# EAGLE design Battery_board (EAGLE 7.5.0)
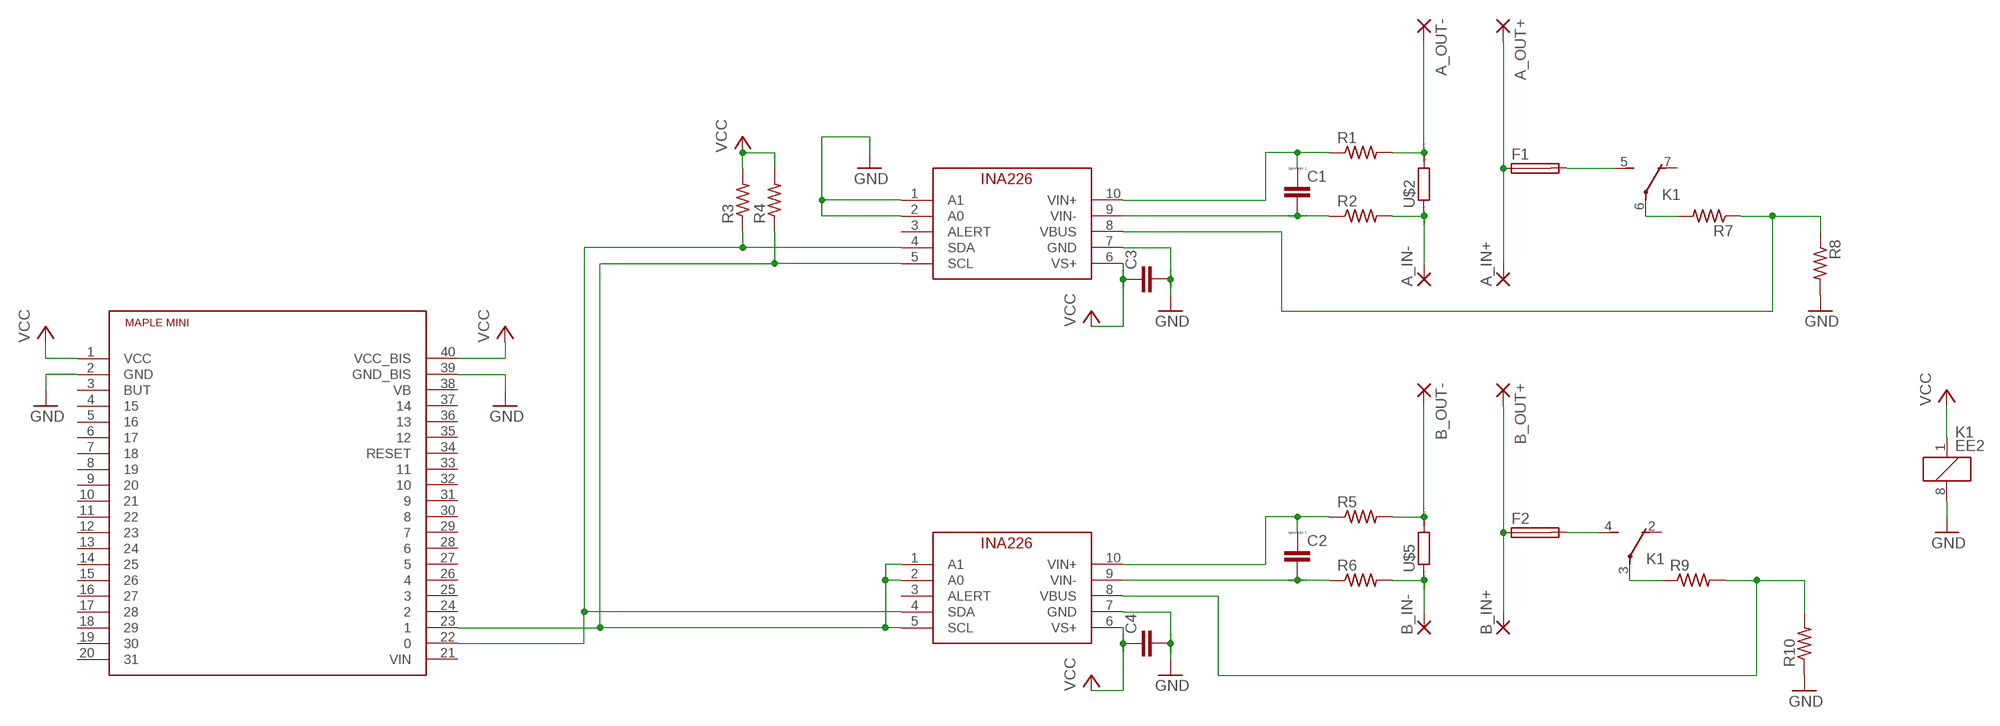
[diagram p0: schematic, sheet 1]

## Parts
A_IN+  WIREPAD4,16O1,6  [4,16O1,6]
A_IN-  WIREPAD4,16O1,6  [4,16O1,6]
A_OUT+  WIREPAD4,16O1,6  [4,16O1,6]
A_OUT-  WIREPAD4,16O1,6  [4,16O1,6]
B_IN+  WIREPAD4,16O1,6  [4,16O1,6]
B_IN-  WIREPAD4,16O1,6  [4,16O1,6]
B_OUT+  WIREPAD4,16O1,6  [4,16O1,6]
B_OUT-  WIREPAD4,16O1,6  [4,16O1,6]
C1  CC0603  [C0603]
C2  CC0603  [C0603]
C3  CC0603  [C0603]
C4  CC0603  [C0603]
F1  TE5  [TE5]
F2  TE5  [TE5]
K1  EE2  [EE2-5NU]
R1  R-US_R0603  [R0603]
R2  R-US_R0603  [R0603]
R3  R-US_R0603  [R0603]
R4  R-US_R0603  [R0603]
R5  R-US_R0603  [R0603]
R6  R-US_R0603  [R0603]
R7  R-US_R1206  [R1206]
R8  R-US_R1206  [R1206]
R9  R-US_R1206  [R1206]
R10  R-US_R1206  [R1206]
U$1  INA226  [MSOP10]
U$2  R_SHUNT_2526  [R2526]
U$3  MAPLE_MINI  [DIL40_MAPLE]
U$4  INA226  [MSOP10]
U$5  R_SHUNT_2526  [R2526]

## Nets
GND: C3.2 C4.2 K1.8 R8.2 R10.1 U$1.1(A1) U$1.2(A0) U$1.7(GND) U$3.2(GND) U$3.39(GND_BIS) U$4.7(GND)
N$1: R4.1 U$1.5(SCL) U$3.23 U$4.1(A1) U$4.2(A0) U$4.5(SCL)
N$2: C1.1 R1.1 U$1.10(VIN+)
N$3: C1.2 R2.1 U$1.9(VIN-)
N$4: F1.2 K1.5(3:S)
N$7: A_OUT-.1(P) R1.2 U$2.2
N$8: A_IN-.1(P) R2.2 U$2.1
N$9: A_IN+.1(P) A_OUT+.1(P) F1.1
N$10: F2.2 K1.4(2:S)
N$12: C2.1 R5.1 U$4.10(VIN+)
N$13: C2.2 R6.1 U$4.9(VIN-)
N$16: R3.1 U$1.4(SDA) U$3.22 U$4.4(SDA)
N$18: B_OUT-.1(P) R5.2 U$5.2
N$19: B_IN-.1(P) R6.2 U$5.1
N$20: B_IN+.1(P) B_OUT+.1(P) F2.1
N$21: K1.3(2:P) R9.1
N$22: R9.2 R10.2 U$4.8(VBUS)
N$23: K1.6(3:P) R7.2
N$24: R7.1 R8.1 U$1.8(VBUS)
VCC: C3.1 C4.1 K1.1 R3.2 R4.2 U$1.6(VS+) U$3.1(VCC) U$3.40(VCC_BIS) U$4.6(VS+)
Unconnected: K1.2(2:O) K1.7(3:O) U$1.3(ALERT) U$3.3(BUT) U$3.4 U$3.5 U$3.6 U$3.7 U$3.8 U$3.9 U$3.10 U$3.11 U$3.12 U$3.13 U$3.14 U$3.15 U$3.16 U$3.17 U$3.18 U$3.19 U$3.20 U$3.21(VIN) U$3.24 U$3.25 U$3.26 U$3.27 U$3.28 U$3.29 U$3.30 U$3.31 U$3.32 U$3.33 U$3.34(RESET) U$3.35 U$3.36 U$3.37 U$3.38(VB) U$4.3(ALERT)

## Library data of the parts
A_IN+ A_IN- A_OUT+ A_OUT- B_IN+ B_IN- B_OUT+ B_OUT- = wirepad:WIREPAD: Wire PAD connect wire on PCB
C1-C4 = eagle-ltspice:C: CAPACITOR, European symbol; SPICEMODEL: NONE; SPICEPREFIX: C
F1 F2 = fuse:TE5: FUSE; OC_FARNELL: unknown; OC_NEWARK: unknown
K1 = CUSTOM:EE2: Compact & Slim 2 Form C Non-polarized Relay NAiS Source: http://www.mew-europe.com/.. en_ds_61011_0000.pdf
R1-R10 = resistor:R-US_: RESISTOR, American symbol
U$1 U$4 = CUSTOM:INA226: INA226
U$2 U$5 = CUSTOM:R_SHUNT_2526
U$3 = CUSTOM:MAPLE_MINI

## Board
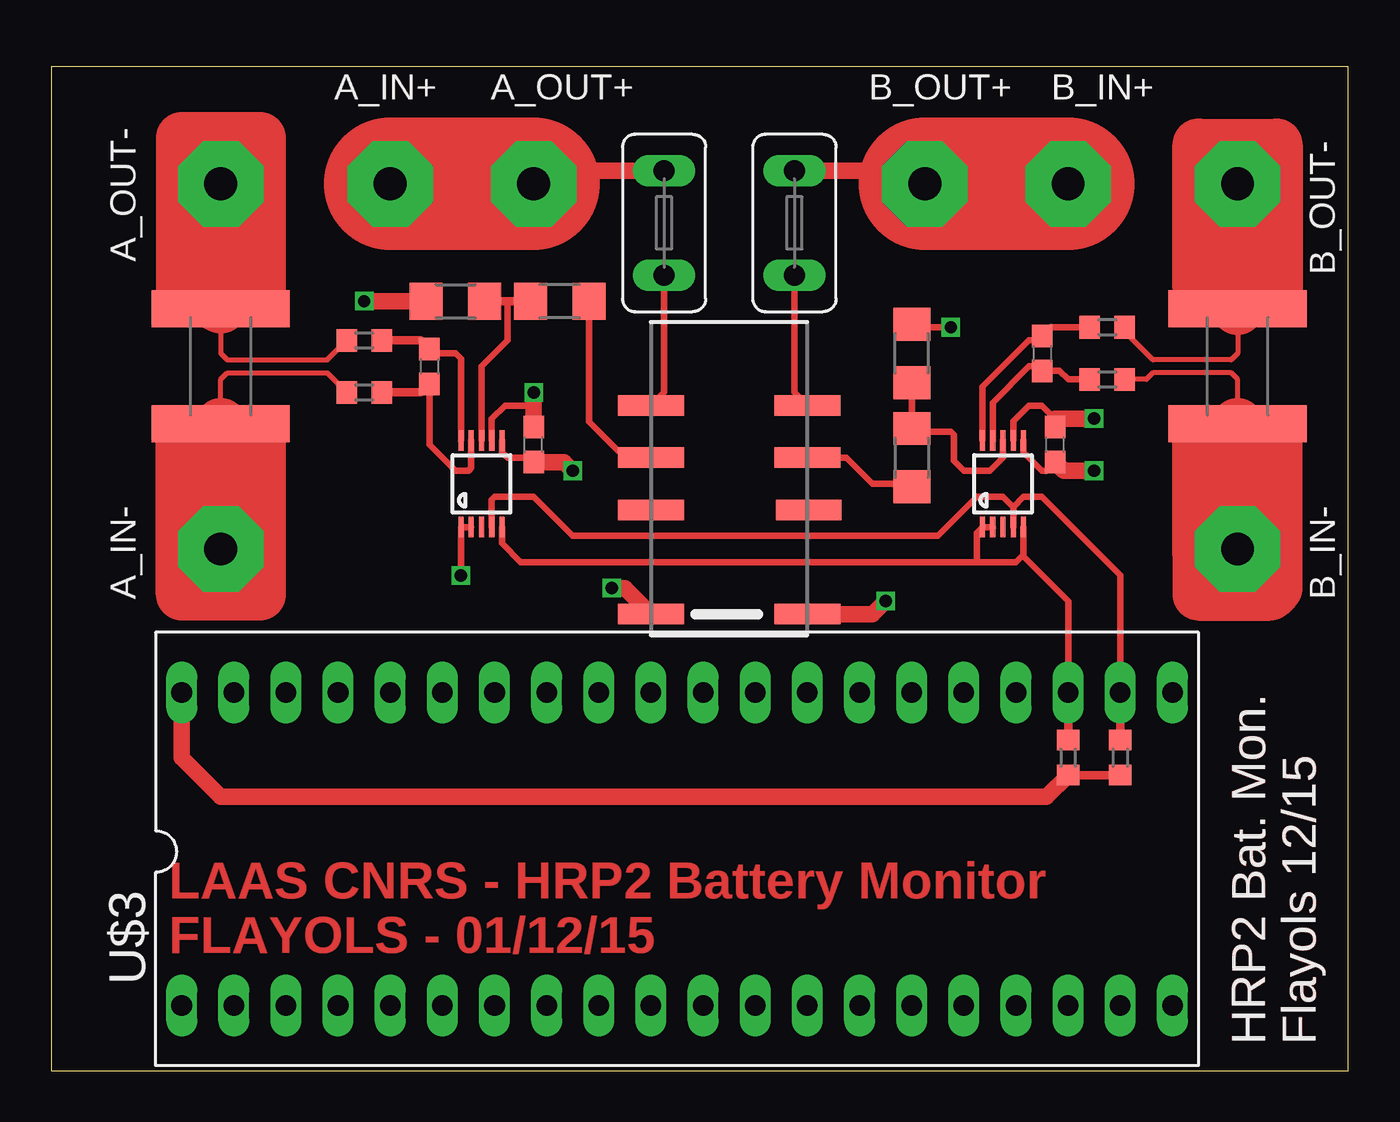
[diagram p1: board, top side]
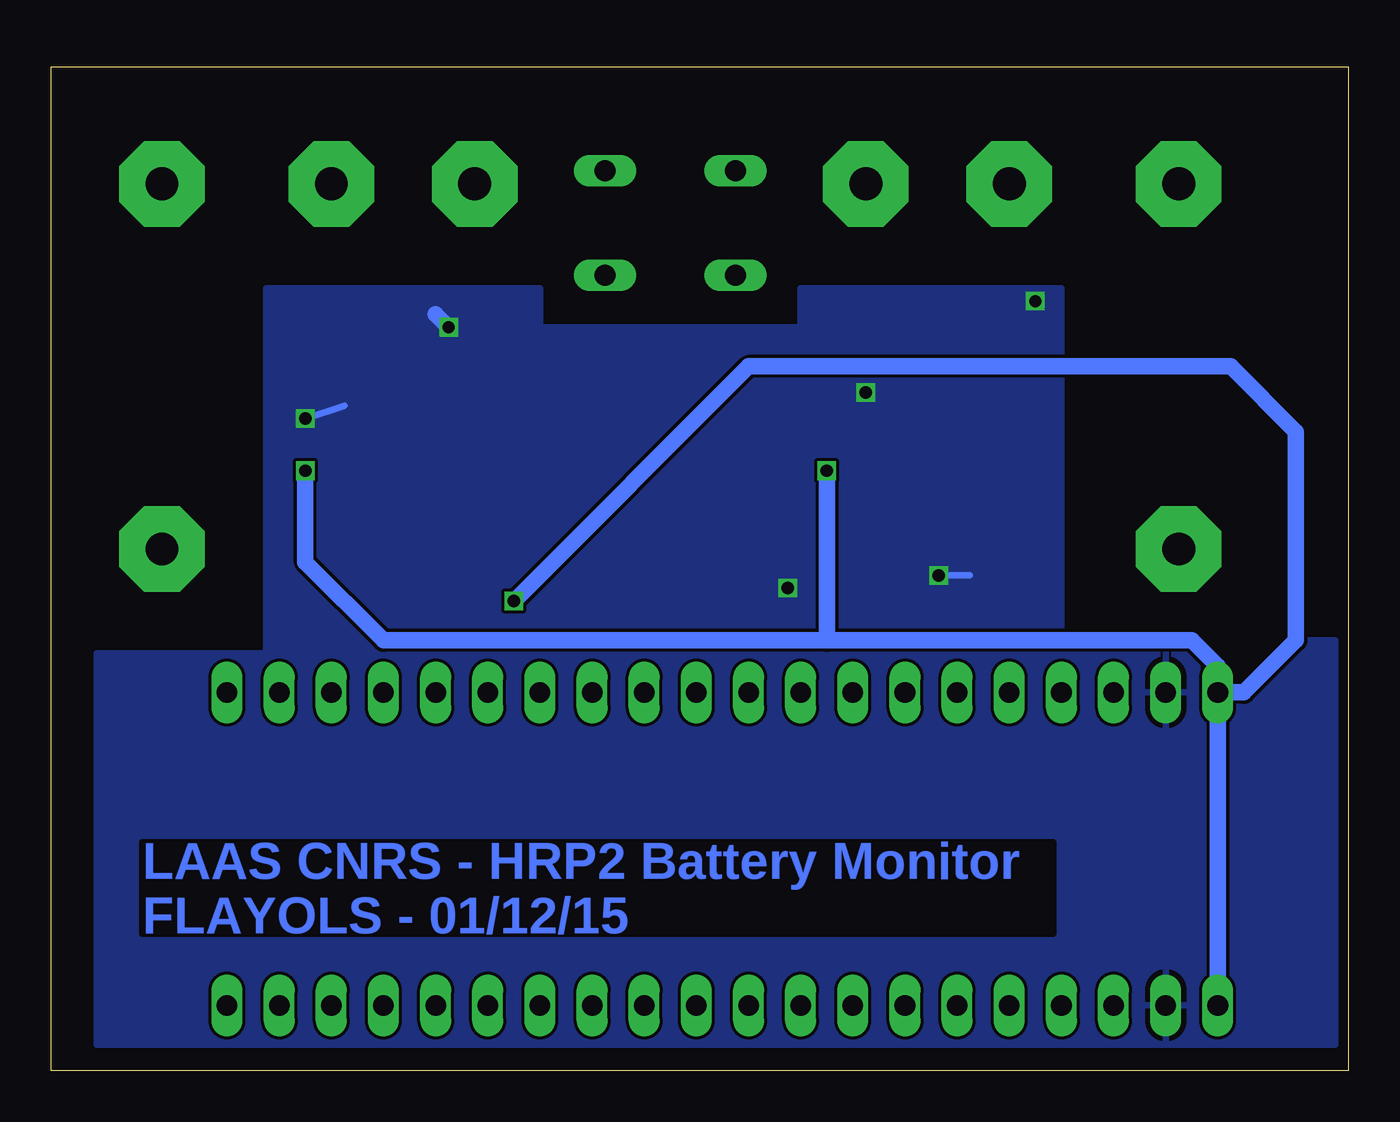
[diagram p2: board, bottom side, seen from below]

Size 63.17 x 48.88 mm. Coordinates in mm from the lower left corner, seen from the top.
Outline: 0,0 63.17,0 63.17,48.88 0,48.88 0,0
Copper layers (1*16): Top 0.035mm / dielectric 1.5mm / Bottom 0.035mm
Design rules "SeeedStudio_2layer_DRU_no_angle_20140221": minimum track width 6mil, minimum drill 12mil, track to track 6mil, track to pad 6mil, pad to pad 6mil, via to via 6mil, smd to smd 0mil, copper to edge 10mil, drill to drill 10mil, minimum pad ring 10mil, minimum via ring 6mil, stop-mask expansion 2mil, vias tented up to drill 100mil, thermal gap 10mil

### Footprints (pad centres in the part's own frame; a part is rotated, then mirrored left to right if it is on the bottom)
4,16O1,6 = drill 1.6 pad 4.166 octagon: 1 0,0
C0603 = smd 1.1 x 1: 1 -0.85,0; 2 0.85,0
TE5 = drill 1.016 long: 1 -2.54,0; 2 2.54,0
EE2-5NU = smd 1 x 3.2: 1 -5.08,-5.08; 2 0,-5.14; 3 2.54,-5.08; 4 5.08,-5.08; 5 5.08,2.54; 6 2.54,2.54; 7 0,2.54; 8 -5.08,2.54
R0603 = smd 1 x 1.1: 1 -0.85,0; 2 0.85,0
R1206 = smd 1.6 x 1.803: 1 -1.422,0; 2 1.422,0
MSOP10 = smd 0.25 x 1: 1 -1,-2.113; 2 -0.5,-2.113; 3 0,-2.113; 4 0.5,-2.113; 5 1,-2.113; 6 1,2.113; 7 0.5,2.113; 8 0,2.113; 9 -0.5,2.113; 10 -1,2.113
R2526 = smd 1.8 x 6.731: 1 -2.8,0; 2 2.8,0
DIL40_MAPLE = drill 1 long: 1 -24.13,-7.62; 2 -21.59,-7.62; 3 -19.05,-7.62; 4 -16.51,-7.62; 5 -13.97,-7.62; 6 -11.43,-7.62; 7 -8.89,-7.62; 8 -6.35,-7.62; 9 -3.81,-7.62; 10 -1.27,-7.62; 11 1.27,-7.62; 12 3.81,-7.62; 13 6.35,-7.62; 14 8.89,-7.62; 15 11.43,-7.62; 16 13.97,-7.62; 17 16.51,-7.62; 18 19.05,-7.62; 19 21.59,-7.62; 20 24.13,-7.62; 21 24.13,7.62; 22 21.59,7.62; 23 19.05,7.62; 24 16.51,7.62; 25 13.97,7.62; 26 11.43,7.62; 27 8.89,7.62; 28 6.35,7.62; 29 3.81,7.62; 30 1.27,7.62; 31 -1.27,7.62; 32 -3.81,7.62; 33 -6.35,7.62; 34 -8.89,7.62; 35 -11.43,7.62; 36 -13.97,7.62; 37 -16.51,7.62; 38 -19.05,7.62; 39 -21.59,7.62; 40 -24.13,7.62

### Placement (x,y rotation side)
A_IN+  16.51,43.18 0 top
A_IN-  8.25,25.4 270 top
A_OUT+  23.5,43.18 0 top
A_OUT-  8.25,43.18 270 top
B_IN+  49.53,43.18 0 top
B_IN-  57.78,25.4 270 top
B_OUT+  42.55,43.18 0 top
B_OUT-  57.78,43.18 270 top
C1  18.41,34.29 270 top
C2  48.26,34.92 270 top
C3  23.5,30.48 90 top
C4  48.9,30.48 90 top
F1  29.84,41.27 270 top
F2  36.2,41.27 270 top
K1  31.75,27.3 90 top
R1  15.24,35.56 180 top
R2  15.24,33.02 180 top
R3  52.07,15.24 270 top
R4  49.53,15.24 270 top
R5  51.44,36.2 0 top
R6  51.44,33.66 0 top
R7  24.77,37.47 0 top
R8  19.68,37.47 180 top
R9  41.91,29.84 90 top
R10  41.91,34.92 270 top
U$1  20.95,28.57 0 top
U$2  8.25,34.29 90 top
U$3  30.48,10.79 0 top
U$4  46.35,28.57 0 top
U$5  57.78,34.29 90 top

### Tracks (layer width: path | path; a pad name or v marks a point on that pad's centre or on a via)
GND  (via drill 0.6)
  Top 0.305: U$4.7 46.85,31.61 47.62,32.38 48.26,32.38 48.9,31.75 C4.2 | U$1.7 21.45,31.75 22.09,32.38 23.5,32.38 | U$1.2 U$1.1 v19.95,24.11 | R10.1 41.91,36.2 v43.81,36.2
  Top 0.813: R8.2 v15.24,37.47 | 48.9,31.75 v50.8,31.75 | v27.3,23.5 27.94,23.5 K1.8 | C3.2 23.5,32.38 v23.5,33.02
  Bottom 0.305: 48.9,32.38 v50.8,31.75 | v19.95,24.11 19.93,24.13 18.41,24.13
  Bottom 0.813: v43.81,36.2 44.45,36.83
  pour Bottom: 13.97,20.95 13.97,38.1 26.67,38.1 26.67,36.2 39.37,36.2 39.37,38.1 52.7,38.1 52.7,20.32 60.96,20.32 60.96,1.27 0.63,1.27 0.63,20.95
N$1
  Top 0.305: U$1.5 21.95,25.67 22.86,24.77 45.09,24.77 | 45.09,24.77 45.09,26.19 U$4.1 U$4.2 | U$3.23 49.53,22.86 47.35,25.04 47.35,25.13 | U$4.5 47.35,25.13 | 47.35,25.13 46.99,24.77 45.09,24.77
  Top 0.406: U$3.23 R4.1
N$2
  Top 0.305: U$1.10 19.95,34.66 19.68,34.92 18.63,34.92 C1.1
  Top 0.406: R1.1 18,35.56 C1.1
N$3
  Top 0.305: U$1.9 20.45,29.34 20.32,29.21 19.68,29.21 18.41,30.48 C1.2
  Top 0.406: R2.1 18,33.02 C1.2
N$4
  Top 0.305: F1.2 29.84,33.02 K1.5
N$7
  Top 0.254: 8.25,37.15 U$2.2 8.25,34.92 8.57,34.61 13.44,34.61 R1.2
  Top 0.406: 8.25,38.1 10.16,37.09 8.89,37.09 U$2.2 | R1.2 14.39,35.34
  Top 1.778: 10.16,37.78 8.89,38.1 8.89,37.09
  Top 2.54: 6.35,45.4 A_OUT-.1 8.25,37.15 7.62,37.47 6.35,37.47 6.35,45.4 | 10.16,37.78 10.16,45.4 6.35,45.4
N$8
  Top 0.254: U$2.1 8.25,33.66 8.57,33.97 13.44,33.97 R2.2
  Top 0.406: R2.2 14.39,33.23
  Top 2.54: A_IN-.1 6.98,25.4 6.35,23.18 | 6.35,23.18 6.35,31.11 8.25,31.11 | 8.89,30.48 8.25,31.11 | 8.25,31.11 A_IN-.1 | A_IN-.1 10.16,23.18 | 10.16,31.11 10.16,23.18 | 10.16,23.18 6.35,23.18 | 6.35,23.18 8.25,25.08 U$2.1
N$9
  Top 0.813: F1.1 24.13,43.81 A_OUT+.1
  Top 6.452: A_IN+.1 A_OUT+.1
N$10
  Top 0.305: F2.2 36.2,33.02 K1.4
N$12
  Top 0.305: R5.1 48.68,36.2 C2.1 48.05,35.56 47.62,35.56 45.35,33.29 U$4.10
N$13
  Top 0.305: U$4.9 45.85,32.52 47.62,34.29 48.05,34.29 C2.2 49.11,34.08 49.53,33.66 R6.1
N$16
  Top 0.305: U$1.4 21.45,27.8 21.59,27.94 23.5,27.94 25.4,26.04 43.18,26.04 45.09,27.94 46.35,27.94 46.85,27.44 | U$3.22 52.07,24.13 48.26,27.94 47.35,27.94 46.85,27.44 | 46.85,27.44 U$4.4
  Top 0.406: U$3.22 R3.1
N$18
  Top 0.254: 55.88,38.1 57.78,36.2 57.78,34.92 57.47,34.61 53.66,34.61 52.28,35.98 R5.2
  Top 2.54: 55.88,38.1 55.88,45.09 59.69,45.09 59.69,37.78 57.78,40.01 B_OUT-.1 U$5.2
N$19
  Top 0.254: 57.78,31.11 U$5.1 57.78,33.66 57.47,33.97 53.66,33.97 53.34,33.66 R6.2 | 55.88,31.11 56.26,31.49
  Top 2.54: 57.78,24.13 B_IN-.1 57.78,27.62 57.78,29.21 | 57.78,24.13 57.78,23.18 55.88,25.08 | 55.88,25.08 55.88,23.5 | 55.88,23.5 55.88,23.18 59.37,23.18 59.69,23.5 59.69,31.11 57.78,29.21 | 57.78,24.13 57.15,23.5 55.88,23.5 | 55.88,25.08 55.88,31.11 | U$5.1 57.78,29.21
N$20
  Top 0.813: 42.55,44.45 B_OUT+.1 41.91,43.81 F2.1
  Top 6.452: B_OUT+.1 B_IN+.1
N$21
  Top 0.305: K1.3 38.73,29.84 40.01,28.57 41.76,28.57 R9.1
N$22
  Top 0.305: U$4.8 46.35,29.84 45.72,29.21 44.45,29.21 43.97,29.69 43.97,30.96 43.81,31.11 42.06,31.11 R9.2 R10.2
N$23
  Top 0.305: R7.2 26.19,31.6 27.94,29.84 K1.6
N$24
  Top 0.305: U$1.8 20.95,34.29 22.23,35.56 22.23,37.47
  Top 0.406: R7.1 22.23,37.47 R8.1
VCC  (via drill 0.6)
  Top 0.305: U$4.6 47.35,30.11 48.26,29.21 48.48,29.21 C4.1 | C3.1 23.28,29.84 22.23,29.84 21.95,30.11 U$1.6
  Top 0.406: R4.2 R3.2
  Top 0.813: R4.2 48.48,13.34 8.25,13.34 6.35,15.24 U$3.40 | v25.4,29.21 24.98,29.63 C3.1 | C4.1 49.31,29.21 v50.8,29.21 | K1.1 40.01,22.23 v40.64,22.86
  Bottom 0.813: U$3.40 U$3.1 | 25.4,20.95 7.62,20.95 6.35,19.68 U$3.40 | 25.4,20.95 46.99,20.95 50.8,24.77 v50.8,29.21 | U$3.40 5.08,18.41 2.54,20.95 2.54,31.11 5.71,34.29 29.21,34.29 v40.64,22.86 | v25.4,29.21 25.4,20.95

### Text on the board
Top: LAAS CNRS - HRP2 Battery Monitor / FLAYOLS - 01/12/15 | HRP2 Bat. Mon. / Flayols 12/15 | HRP2 Bat. Mon. / Flayols 12/15
Bottom: LAAS CNRS - HRP2 Battery Monitor / FLAYOLS - 01/12/15
tPlace: HRP2 Bat. Mon. / Flayols 12/15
